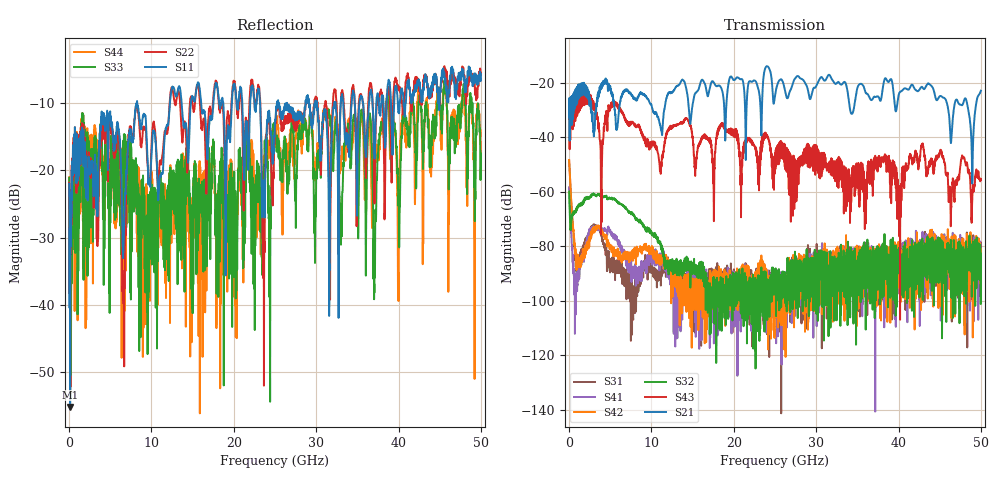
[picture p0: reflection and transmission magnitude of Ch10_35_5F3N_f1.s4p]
!Agilent Technologies,N5247A,US51170199,A.09.90.13
!Agilent N5247A: A.09.90.13
!Date: Wednesday, December 16, 2015 12:34:19
!Correction: S11(Full 4 Port(1,2,3,4))
!S12(Full 4 Port(1,2,3,4))
!S13(Full 4 Port(1,2,3,4))
!S14(Full 4 Port(1,2,3,4))
!S21(Full 4 Port(1,2,3,4))
!S22(Full 4 Port(1,2,3,4))
!S23(Full 4 Port(1,2,3,4))
!S24(Full 4 Port(1,2,3,4))
!S31(Full 4 Port(1,2,3,4))
!S32(Full 4 Port(1,2,3,4))
!S33(Full 4 Port(1,2,3,4))
!S34(Full 4 Port(1,2,3,4))
!S41(Full 4 Port(1,2,3,4))
!S42(Full 4 Port(1,2,3,4))
!S43(Full 4 Port(1,2,3,4))
!S44(Full 4 Port(1,2,3,4))
!S4P File: Measurements: <S11,S12,S13,S14>,
!<S21,S22,S23,S24>,
!<S31,S32,S33,S34>,
!<S41,S42,S43,S44>:
# Hz S  dB  R 50
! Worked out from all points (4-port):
!   3201 points, 10 MHz to 50 GHz, reference 50 ohm
!   strongest paths, dB at 10 MHz, 12.51 GHz, 25 GHz, 37.5 GHz, 50 GHz:
!     S21: -32.5, -23.4, -25.0, -24.9, -22.8
!     S43: -33.2, -35.7, -45.8, -47.7, -55.4
!     S32: -59.8, -88.7, -89.1, -80.2, -83.1
!     S42: -48.2, -88.8, -98.9, -86.3, -88.3
!     S41: -58.3, -88.0, -92.3, -89.6, -85.6
!     S31: -48.3, -89.7, -93.5, -91.2, -81.5
!   lowest |S11| = -55.2 dB at 135 MHz (marker M1), VSWR 1.00, Z = 50 + j0.172 ohm
!   |S11| at or under -10 dB: start of sweep to 8.229 GHz; 8.279 GHz to 12.26 GHz (3.98 GHz wide, 38.8 % of centre); 26.46 GHz to 28.71 GHz (2.242 GHz wide, 8.13 % of centre)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
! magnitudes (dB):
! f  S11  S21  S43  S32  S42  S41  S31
! 10 MHz  -22.0  -32.5  -33.2  -59.8  -48.2  -58.3  -48.3
! 135 MHz  -55.2  -32.7  -32.7  -72.2  -55.8  -68.2  -55.7
! 916.1 MHz  -18.0  -26.6  -32.2  -66.2  -88.7  -92.9  -85.4
! 6.634 GHz  -30.7  -23.3  -31.6  -65.3  -83.1  -81.2  -90.4
! 8.18 GHz  -10.0  -26.2  -36.2  -69.6  -83.6  -90.4  -97.6
! 23.63 GHz  -23.0  -17.3  -40.4  -98.5  -89.4  -89.6  -108.8
! 50 GHz  -5.6  -22.8  -55.4  -83.1  -88.3  -85.6  -81.5
